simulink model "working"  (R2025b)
settings: Solver=FixedStepAuto  StartTime=0.0  StopTime=inf  RelTol=1e-3
undefined symbols (not defined in the file or in its folder): servoAngle, targetAngle
libraries: arduinolib x4, slpidlib x1

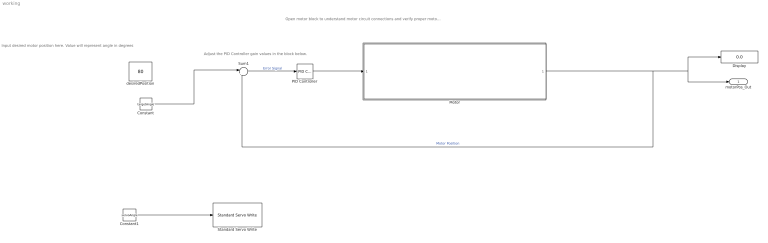
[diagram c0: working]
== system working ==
  note: Adjust the PID Controller gain values in the block below.
  note: Input desired motor position here. Value will represent angle in degrees
  note: Open motor block to understand motor circuit connections and verify proper motor encoder functionality.
  Constant : Constant  Value=targetAngle
  Constant1 : Constant  Value=servoAngle
  Display : Display
  Motor : Subsystem
  PID Controller : slpidlib/PID Controller  Controller=PID  Form=Parallel  TimeDomain=Continuous-time  UseExternalTs=off  SampleTime=-1  IntegratorMethod=Forward Euler  FilterMethod=Forward Euler  ControllerParametersSource=internal  P=0.5  I=0  UseKiTs=off  D=0.01  UseExternalDerivativeSource=off  N=200  UseFilter=on  TunerSelectOption=Transfer Function Based (PID Tuner App)  InitialConditionSource=internal  InitialConditionForIntegrator=0  InitialConditionForFilter=0  DifferentiatorICPrevScaledInput=0  ExternalReset=none  TrackingMode=off  Kt=1  LimitOutput=off  SatLimitsSource=internal  UpperSaturationLimit=inf  LowerSaturationLimit=-inf  LinearizeAsGain=on  AntiWindupMode=none  Kb=1  LimitIntegrator=off  UpperIntegratorSaturationLimit=inf  LowerIntegratorSaturationLimit=-inf  POutMin=[]  POutMax=[]  IOutMin=[]  IOutMax=[]  DOutMin=[]  DOutMax=[]  NOutMin=[]  NOutMax=[]  SumOutMin=[]  SumOutMax=[]  SaturationOutMin=[]  SaturationOutMax=[]  PParamMin=[]  PParamMax=[]  IParamMin=[]  IParamMax=[]  DParamMin=[]  DParamMax=[]  NParamMin=[]  NParamMax=[]  KbParamMin=[]  KbParamMax=[]  KtParamMin=[]  KtParamMax=[]  KbOutMin=[]  KbOutMax=[]  KtOutMin=[]  KtOutMax=[]  IntegratorOutMin=[]  IntegratorOutMax=[]  FilterOutMin=[]  FilterOutMax=[]  SumI1OutMin=[]  SumI1OutMax=[]  SumI2OutMin=[]  SumI2OutMax=[]  SumI3OutMin=[]  SumI3OutMax=[]  SumI4OutMin=[]  SumI4OutMax=[]  SumDOutMin=[]  SumDOutMax=[]  DifferentiatorOutMin=[]  DifferentiatorOutMax=[]  FilterDiffOutCoefMin=[]  FilterDiffOutCoefMax=[]  ReciprocalOutMin=[]  ReciprocalOutMax=[]  SumDenOutMin=[]  SumDenOutMax=[]  SumNumOutMin=[]  SumNumOutMax=[]  DivideOutMin=[]  DivideOutMax=[]  UdiffTsProdOutMin=[]  UdiffTsProdOutMax=[]  NTsProdOutMin=[]  NTsProdOutMax=[]  UintegralTsProdOutMin=[]  UintegralTsProdOutMax=[]  UngainTsProdOutMin=[]  UngainTsProdOutMax=[]  ClampingZeroOutDataTypeStr=Inherit: Inherit via back propagation  ClampingZeroOutMin=[]  ClampingZeroOutMax=[]  FilterDenConstantOutDataTypeStr=Inherit: Inherit via back propagation  FilterDenConstantOutMin=[]  FilterDenConstantOutMax=[]  PCopyOutDataTypeStr=Inherit: Inherit via back propagation  PCopyOutMin=[]  PCopyOutMax=[]  NCopyOutDataTypeStr=Inherit: Inherit via back propagation  NCopyOutMin=[]  NCopyOutMax=[]  IntegratorContinuousStateAttributes=''  IntegratorStateMustResolveToSignalObject=off  IntegratorRTWStateStorageClass=Auto  FilterContinuousStateAttributes=''  FilterStateMustResolveToSignalObject=off  FilterRTWStateStorageClass=Auto  ParallelPVariant=InternalParameters  IdealPVariant=Disabled  IVariant=InternalParameters  DVariant=InternalParameters  IntegratorVariant=Continuous  SatVariant=Disabled  AWVariant=Passthrough  PCopyVariant=Disabled  TRVariant=Disabled  FdbkBlocksVariant=Forward  IdealPFdbkVariant=Disabled  SatFdbkVariant=Disabled  DerivativeFilterVariant=ContFilter  NVariant=InternalParameters  NCopyVariant=Disabled  FilterICVariant=InternalICsFilter  IntegratorICVariant=InternalICs  ExternalResetVariant=Disabled  TRSumVariant=Passthrough  SumFdbkVariant=Disabled  SumVariant=Sum_PID  TsampFilterVariant=InternalTs  TsampNgainVariant=Passthrough  TsampIntegralVariant=Disabled_SignalSpec  ExternalSaturationOutDataTypeStr=Inherit: Same as second input  DerivativeSourceVariant=ErrorSignal  PreIntVariant=InternalPreInt
  Standard Servo Write : arduinolib/Standard Servo Write  pinNumber=12  ServoIndex=0  blockPlatform=ARDUINO
  Sum1 : Sum  Inputs=|+-
  desiredPosition : Constant  Value=80
  motorPos_Out : Outport  VectorParamsAs1DForOutWhenUnconnected=off
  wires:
  Motor/1(position in degrees) -> motorPos_Out/1, Display/1, Sum1/2  "Motor Position"
  Sum1/1 -> PID Controller/1  "Error Signal"
  PID Controller/1 -> Motor/1(unfiltered control input1)
  Constant/1 -> Sum1/1
  Constant1/1 -> Standard Servo Write/1

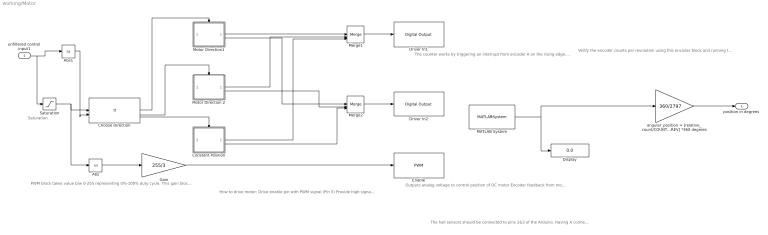
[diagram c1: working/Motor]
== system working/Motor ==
  note: The counter works by triggering an interrupt from encoder A on the rising edge. It then uses the value from encoder B to determine what direction the motor is turning. Review how quadrature encoders use gray code if you're rusty on that!
  note: PWM block takes value b/w 0-255 representing 0%-100% duty cycle. This gain block scales the output voltage based on the error. The motor will move more slowly as the error grows smaller. The scale is based on the thresholds of the saturation block.
  note: Outputs analog voltage to control position of DC motor Encoder feedback from motor calculated using interrupt pins on the Arduino Helpful (but not necessary) to convert encoder ticks to degrees using the gain block
  note: Saturation
  note: How to drive motor: Drive enable pin with PWM signal (Pin 5) Provide high signal to IN pin on motor driver Provide low signal to following IN pin on the motor driver Example: Connect pins 30&31 to IN1 and IN2 on motor driver Driving pin 30 high and pin 31 low will cause the motor to spin one direction Reversing pins 30 and 31 will cause the motor to spin the other direction
  note: The hall sensors should be connected to pins 2&3 of the Arduino. Having A connected to pin 2 and B connected to pin 3 will spin the motor one way, and reversing them will spin the motor the opposite way.
  note: Verify the encoder counts per revolution using this encoder block and running the model. Adjustments may need to be made to the current value (2797)
  unfiltered control input1 : Inport
  Abs : Abs
  Abs1 : Abs
  Choose Direction : If  NumInputs=2  IfExpression=u1 > 0 & u2 > 3  ElseIfExpressions=u1 < 0 & u2 > 3
  Constant Position : Subsystem  TreatAsAtomicUnit=on
  Display : Display
  Driver In1 : arduinolib/Digital Output  pinNumber=30  Direction=output  blockPlatform=arduino
  Driver In2 : arduinolib/Digital Output  pinNumber=31  Direction=output  blockPlatform=arduino
  Enable : arduinolib/PWM  pinNumber=5  frequencyType=Default  desiredFrequency=490.2  achievableFrequency=490.2
  Gain : Gain  Gain=255/3
  MATLAB System : MATLABSystem  System=Encoder_arduino  Encoder=0  PinA=2  PinB=3  SampleTime=0.001
  Merge1 : Merge  Inputs=3
  Merge2 : Merge  Inputs=3
  Motor Direction 2 : Subsystem  TreatAsAtomicUnit=on
  Motor Direction1 : Subsystem  TreatAsAtomicUnit=on
  Saturation : Saturate  UpperLimit=5  LowerLimit=-5
  angular_position = [relative_count/COUNTS_PER_REV] *360 degrees : Gain  Gain=360/2797
  position in degrees : Outport  VectorParamsAs1DForOutWhenUnconnected=off
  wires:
  angular_position = [relative_count/COUNTS_PER_REV] *360 degrees/1 -> position in degrees/1
  Saturation/1 -> Abs/1, Choose Direction/1
  Choose Direction/1 -> Motor Direction1/Action
  Motor Direction1/1(IN1) -> Merge1/1
  Motor Direction 2/1(IN1) -> Merge1/2
  Motor Direction1/2(IN2) -> Merge2/1
  Motor Direction 2/2(IN2) -> Merge2/2
  Abs/1 -> Gain/1
  Gain/1 -> Enable/1
  Merge1/1 -> Driver In1/1
  Merge2/1 -> Driver In2/1
  Constant Position/2(IN2) -> Merge2/3
  Constant Position/1(IN1) -> Merge1/3
  unfiltered control input1/1 -> Saturation/1, Abs1/1
  Abs1/1 -> Choose Direction/2
  Choose Direction/3 -> Constant Position/Action
  Choose Direction/2 -> Motor Direction 2/Action
  MATLAB System/1 -> Display/1, angular_position = [relative_count/COUNTS_PER_REV] *360 degrees/1

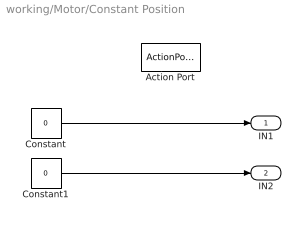
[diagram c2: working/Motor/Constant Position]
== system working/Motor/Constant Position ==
  Action Port : ActionPort  ActionPortLabel=else
  Constant : Constant  Value=0
  Constant1 : Constant  Value=0
  IN1 : Outport
  IN2 : Outport  Port=2
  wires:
  Constant/1 -> IN1/1
  Constant1/1 -> IN2/1

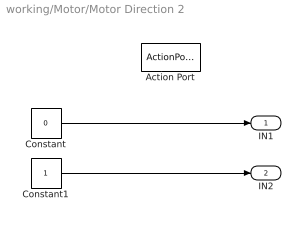
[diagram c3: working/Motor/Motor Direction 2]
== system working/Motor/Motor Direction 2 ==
  Action Port : ActionPort  ActionPortLabel=elseif(u1 < 0 & u2 > 3)
  Constant : Constant  Value=0
  Constant1 : Constant
  IN1 : Outport
  IN2 : Outport  Port=2
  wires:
  Constant/1 -> IN1/1
  Constant1/1 -> IN2/1

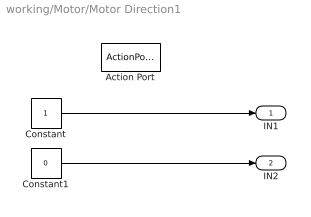
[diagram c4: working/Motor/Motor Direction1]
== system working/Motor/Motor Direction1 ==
  Action Port : ActionPort  ActionPortLabel=if(u1 > 0 & u2 > 3)
  Constant : Constant
  Constant1 : Constant  Value=0
  IN1 : Outport
  IN2 : Outport  Port=2
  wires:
  Constant/1 -> IN1/1
  Constant1/1 -> IN2/1
